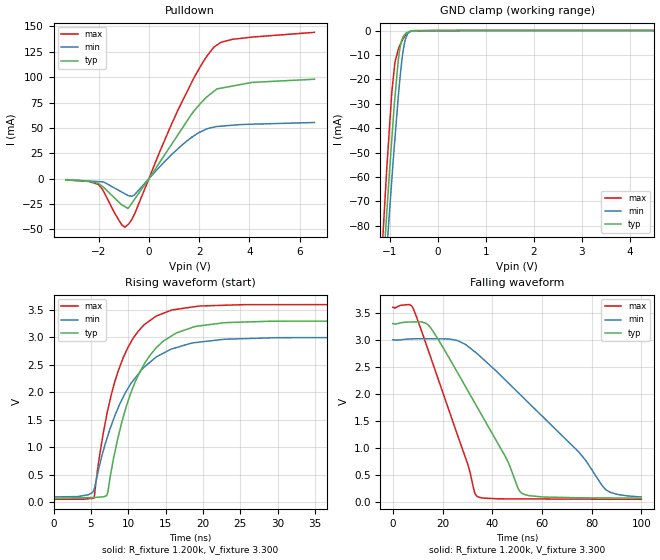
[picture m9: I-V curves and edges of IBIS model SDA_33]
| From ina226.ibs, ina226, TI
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|   SDA Open_drain Model
[Model]   SDA_33
Model_type   I/O_open_drain
Polarity   Non-Inverting
Enable   Active-Low
Vinl = .99
Vinh = 2.31
Vmeas = 1.65
Vref = 1.65
Cref = 2pF
Rref = 1200
|   typ   min   max
|   (nom PVT)   (Fast PVT)   (slow PVT)
|   ON state : BUFFER OUTPUT TURNED HIGH
C_comp   1.201E-12   1.014E-12   1.493E-12
|   OFF state: BUFFER OUTPUT TURNED LOW
|C_comp   9.774E-13   8.711E-13   1.133E-12
| Where   nom PVT is  Nominal Process, 3.3V, 25C
|   Fast PVT is Strong Process, 3.6V, -40C
|   Slow PVT is Weak Process, 3.0V, 85C
|C_comp - from L-C Tank method, L = 1nH, peak frequency
[Model Spec]
| variable   typ   min   max
Vinl   0.99   0.9   1.08
Vinh   2.31   2.1   2.52
|Vinl = 0.3 x V+, Vinh = 0.7 x V+
[Voltage Range]   3.3   3   3.6
|Ambient Temperature Range   27   85   -40
[Temperature Range]   30   88   -40
[Pullup Reference]   3.3   3   3.6
[Pulldown Reference]   0   0   0
[Power Clamp Reference]   3.3   3   3.6
[GND Clamp Reference]   0   0   0
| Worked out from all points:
|   slope of the pulldown table from 0 to 0.495 V, typ, clamps not added: 26.7 ohm
|   GND clamp passes 1 mA (typ) near -0.66 V on its own axis
|   falling waveform, R_fixture 1.200k, V_fixture 3.300: 20-80 % time 23.8ns typ, 37.3ns min, 16.1ns max; typ from 3.3 V to 0.07 V
|   rising waveform, R_fixture 1.200k, V_fixture 3.300: 20-80 % time 4.89ns typ, 5.69ns min, 4.19ns max; typ from 0.07 V to 3.3 V
[Pulldown]
|   Voltage   I(typ)   I(min)   I(max)
-3.3V     -1.186mA   -808.7uA   -1.248mA
-1.997V   -4.922mA   -2.89mA    -5.83mA
-1.089V   -25.49mA   -12.99mA   -45.15mA
-957.3mV  -27.44mA   -14.79mA   -47.72mA
-827.1mV  -29.37mA   -16.57mA   -45.2mA
-586.8mV  -20.85mA   -16.19mA   -35.64mA
1.178V    44.03mA    29.93mA    68.66mA
1.863V    68.63mA    43.41mA    102.4mA
2.588V    86.1mA     50.81mA    129.6mA
3.312V    91.2mA     52.63mA    137.2mA
4.109V    94.84mA    53.69mA    139.5mA
6.59V     97.96mA    55.35mA    144.2mA
[GND Clamp]
|   Voltage   I(typ)   I(min)   I(max)
-3.3V     -809.1mA   -770.2mA   -892.6mA
-1.184V   -110.2mA   -123.5mA   -96.51mA
-1.085V   -80.25mA   -94.98mA   -62.59mA
-1.07V    -75.63mA   -90.72mA   -57.35mA
-1.023V   -61.35mA   -77.85mA   -43.35mA
-957.3mV  -43.2mA    -59.93mA   -24.36mA
-896.9mV  -27.32mA   -44.36mA   -13.01mA
-827.1mV  -12.09mA   -27.14mA   -7.758mA
-781.9mV  -6.039mA   -17.63mA   -5.56mA
-732.5mV  -2.819mA   -9.216mA   -3.536mA
-659mV    -905.4uA   -2.543mA   -1.442mA
6.59V     0A         0A         0A
[POWER Clamp]
|   SCR cell for ESD function. Effects occurr above VDD x 2
|   Voltage   I(typ)   I(min)   I(max)
-3.3V     0A         0A         0A
0V        0A         0A         0A
6.6V      0A         0A         0A
[Ramp]
R_load = 1200
|   typ   min   max
dV/dt_r   1.93818/4.88739e-009   1.717/5.66949e-009   2.13117/4.17272e-009
dV/dt_f   1.93815/2.37856e-008   1.71691/3.73525e-008   2.13116/1.60634e-008
[Falling Waveform]
R_fixture = 1.200k
V_fixture = 3.300
V_fixture_min = 3.000
V_fixture_max = 3.600
C_fixture = 0.000
|  time   V(typ)   V(min)   V(max)
0s        3.3V       3V         3.6V
8.36ns    3.329V     3.017V     3.561V
15.24ns   3.219V     3.018V     2.673V
25.97ns   2.396V     2.986V     1.242V
33.77ns   1.766V     2.748V     107.7mV
45.53ns   815.8mV    2.242V     56.84mV
51.92ns   159.8mV    1.954V     55.81mV
74.83ns   76.92mV    921.6mV    52.11mV
85.57ns   73.85mV    229.7mV    50.38mV
99.93ns   69.74mV    91.64mV    48.06mV
[Rising Waveform]
R_fixture = 1.200k
V_fixture = 3.300
V_fixture_min = 3.000
V_fixture_max = 3.600
C_fixture = 0.000
|  time   V(typ)   V(min)   V(max)
0s        69.7mV     91.64mV    48.06mV
5.391ns   80.94mV    214.8mV    69.17mV
7.126ns   118.8mV    1.147V     1.586V
9.115ns   1.441V     1.854V     2.552V
10.89ns   2.177V     2.253V     3.028V
13ns      2.689V     2.557V     3.316V
15.86ns   3.032V     2.791V     3.5V
19.21ns   3.205V     2.909V     3.567V
29.36ns   3.296V     2.993V     3.597V
99.93ns   3.3V       3V         3.6V
